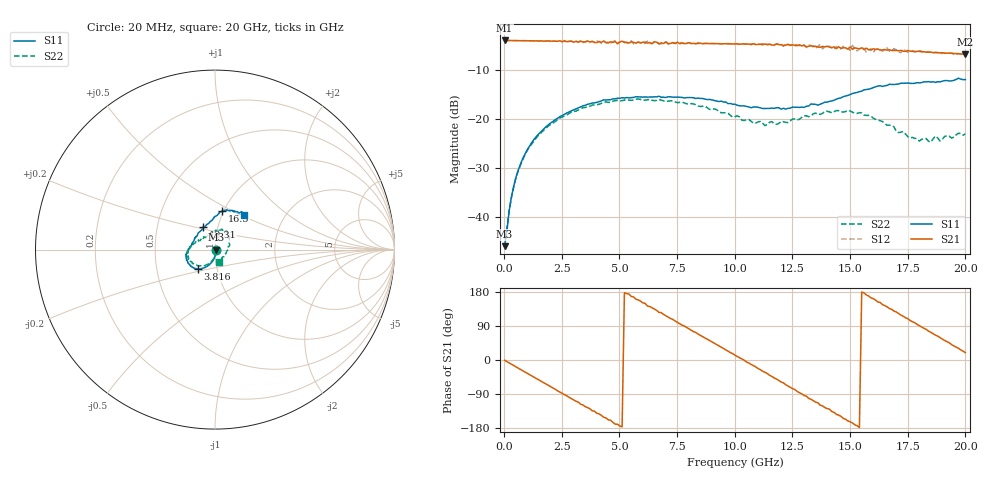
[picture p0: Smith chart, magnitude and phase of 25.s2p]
!Agilent Technologies,N5230A,US43500223,A.07.50.48
!Agilent N5230A: A.07.50.48
!Date: Thursday, September 17, 2015 12:37:23
!Correction: S11(Full 2 Port(1,2))
!S21(Full 2 Port(1,2))
!S12(Full 2 Port(1,2))
!S22(Full 2 Port(1,2))
!S2P File: Measurements: S11, S21, S12, S22:
# Hz S  dB  R 50
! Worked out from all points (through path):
!   201 points, 20 MHz to 20 GHz, reference 50 ohm
!   highest |S21| = -4.07 dB at 20 MHz (marker M1); lowest = -6.9 dB at 20 GHz (marker M2)
!   group delay of S21, straight-line fit = 97.1 ps
!   lowest |S11| = -45.8 dB at 20 MHz (marker M3), VSWR 1.01, Z = 50.5 - j0.121 ohm
!   |S11| at or under -10 dB: start of sweep to end of sweep
!   |S22| runs from -44.3 to -15.9 dB; largest |S21 - S12| = 0.056
!   S11 on the Smith chart (normalised r, x): 20 MHz: 1.01, -0.00; 3.816 GHz: 0.81, -0.18; 13.31 GHz: 0.85, +0.22; 16.5 GHz: 0.99, +0.44; 20 GHz: 1.26, +0.52
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2e7  -45.83 -13.6  -4.07 -0.7  -4.07 -0.7  -44.34 -13.5
4.196e8  -33.53 -77.5  -4.09 -14.9  -4.10 -14.8  -33.75 -79.7
1.019e9  -26.12 -95.5  -4.14 -35.8  -4.14 -35.7  -26.27 -97.1
2.1179e9  -20.51 -112.2  -4.20 -74.3  -4.14 -73.7  -20.83 -116.2
3.4166e9  -17.34 -127.8  -4.34 -118.7  -4.52 -119.6  -17.71 -135.2
3.8162e9  -16.78 -131.8  -4.23 -133.9  -4.30 -133.3  -17.20 -141.7
4.8152e9  -15.92 -143.6  -4.29 -169.2  -4.10 -168.4  -16.29 -155.1
5.5145e9  -15.67 -150.6  -4.36 167.7  -4.14 168.2  -16.22 -162.6
6.7133e9  -15.39 -159.5  -4.78 125.7  -4.69 125.6  -16.03 -173.8
8.012e9  -15.67 -168.2  -4.51 82.3  -4.52 82.8  -17.01 175.5
9.011e9  -16.15 -175.4  -4.67 47.8  -4.73 48.0  -18.05 165.1
1.001e10  -17.01 174.9  -4.78 12.7  -4.69 13.2  -19.53 150.7
1.08092e10  -17.58 166.5  -4.71 -14.9  -4.74 -14.4  -20.88 140.2
1.19081e10  -17.72 148.5  -4.92 -53.9  -4.70 -55.3  -20.93 110.8
1.33067e10  -16.96 118.7  -5.16 -103.6  -5.09 -105.0  -19.33 81.0
1.34066e10  -17.01 117.0  -5.31 -107.3  -5.17 -110.4  -18.95 79.1
1.45055e10  -15.82 97.4  -5.35 -145.5  -5.83 -147.0  -18.32 63.6
1.51049e10  -14.84 91.1  -5.85 -166.3  -5.06 -167.4  -18.63 55.0
1.65035e10  -13.28 79.2  -5.90 143.7  -5.98 145.3  -20.91 28.0
1.67033e10  -12.95 77.4  -5.95 136.0  -6.26 135.8  -21.27 18.9
1.81019e10  -12.61 67.7  -6.37 87.1  -6.20 87.4  -24.15 -36.9
2e10  -12.01 50.5  -6.90 19.6  -6.96 21.1  -23.02 -71.8
